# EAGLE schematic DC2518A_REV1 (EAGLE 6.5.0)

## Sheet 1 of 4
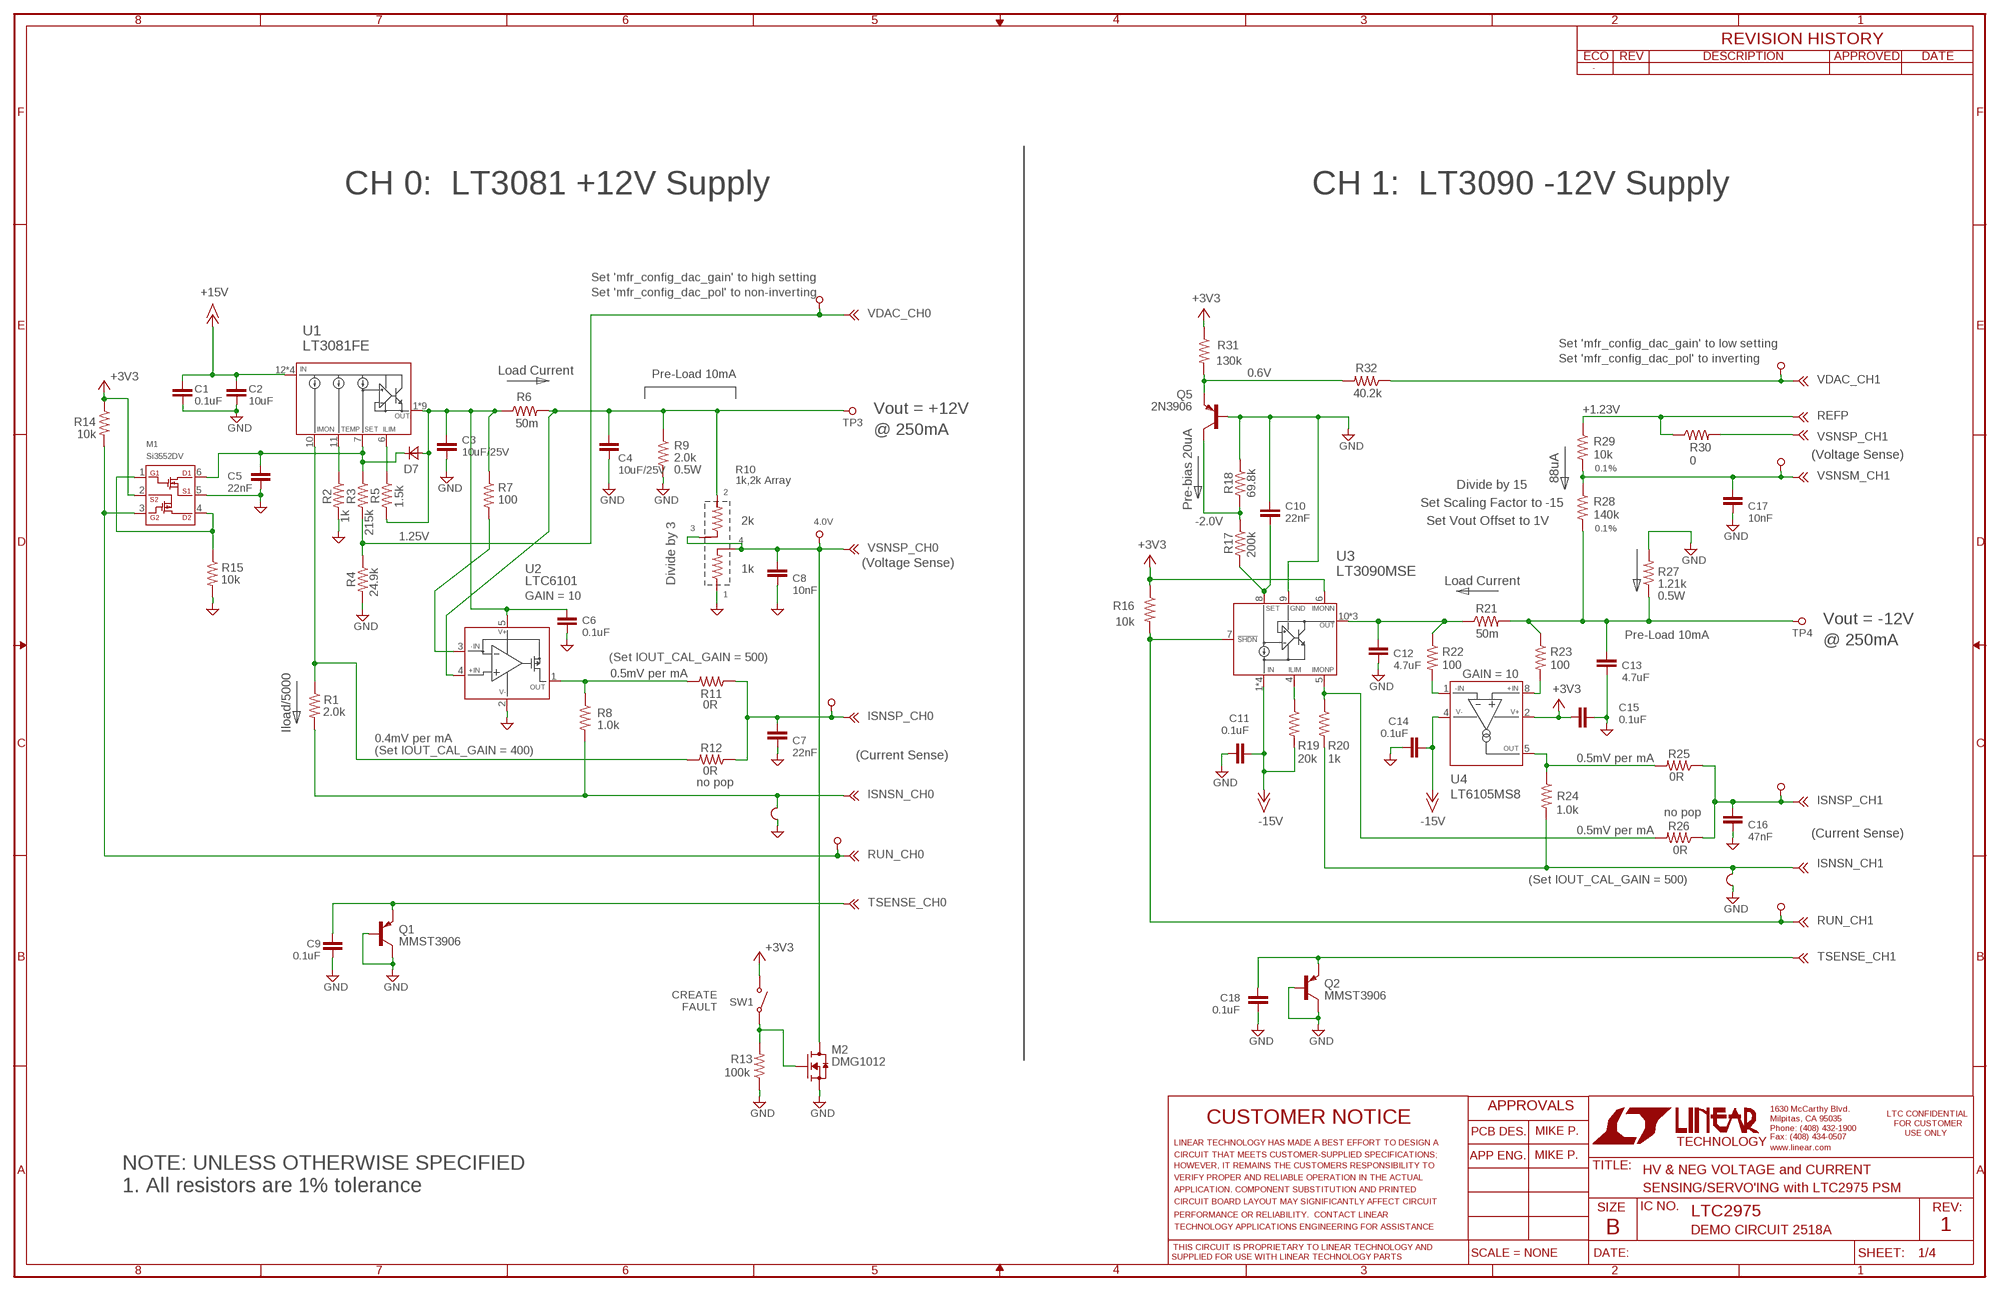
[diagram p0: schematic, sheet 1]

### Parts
C1  0.1uF  CC0603_BOX  [C0603_BOX]
C2  10uF  CC1206_BOX  [C1206_BOX]
C3  10uF/25V  CC1206_BOX  [C1206_BOX]
C4  10uF/25V  CC1206_BOX  [C1206_BOX]
C5  22nF  CC0603_BOX  [C0603_BOX]
C6  0.1uF  CC0603_BOX  [C0603_BOX]
C7  22nF  CC0603_BOX  [C0603_BOX]
C8  10nF  CC0603_BOX  [C0603_BOX]
C9  0.1uF  CC0603_BOX  [C0603_BOX]
C10  22nF  CC0603_BOX  [C0603_BOX]
C11  0.1uF  CC0603_BOX  [C0603_BOX]
C12  4.7uF  CC1206_BOX  [C1206_BOX]
C13  4.7uF  CC1206_BOX  [C1206_BOX]
C14  0.1uF  CC0603_BOX  [C0603_BOX]
C15  0.1uF  CC0603_BOX  [C0603_BOX]
C16  47nF  CC0603_BOX  [C0603_BOX]
C17  10nF  CC0603_BOX  [C0603_BOX]
C18  0.1uF  CC0603_BOX  [C0603_BOX]
D7  DIODE-SOD123  [SOD123]
M1  Si3552DV  NCH-PCH_TS  [TSOP-6]
M2  DMG1012  NCH_SOT323  [SOT323]
Q1  MMST3906  PNPSC  [SC70]
Q2  MMST3906  PNPSC  [SC70]
Q5  2N3906  PNPSOT  [SOT23]
R1  2.0k  RR0603_BOX  [R0603_BOX]
R2  1k  RR0603_BOX  [R0603_BOX]
R3  215k  RR0603_BOX  [R0603_BOX]
R4  24.9k  RR0603_BOX  [R0603_BOX]
R5  1.5k  RR0603_BOX  [R0603_BOX]
R6  50m  RR1210_BOX  [R1210_BOX]
R7  100  RR0603_BOX  [R0603_BOX]
R8  1.0k  RR0603_BOX  [R0603_BOX]
R9  2.0k  RR1210_BOX  [R1210_BOX]
R10  1k,2k Array  R_ARRAY_2X_DIVIDER  [R_ARRAY_2X_ACAS]
R11  0R  RR0603_BOX  [R0603_BOX]
R12  0R  RR0603_BOX  [R0603_BOX]
R13  100k  RR0603_BOX  [R0603_BOX]
R14  10k  RR0603_BOX  [R0603_BOX]
R15  10k  RR0603_BOX  [R0603_BOX]
R16  10k  RR0603_BOX  [R0603_BOX]
R17  200k  RR0603_BOX  [R0603_BOX]
R18  69.8k  RR0603_BOX  [R0603_BOX]
R19  20k  RR0603_BOX  [R0603_BOX]
R20  1k  RR0603_BOX  [R0603_BOX]
R21  50m  RR1210_BOX  [R1210_BOX]
R22  100  RR0603_BOX  [R0603_BOX]
R23  100  RR0603_BOX  [R0603_BOX]
R24  1.0k  RR0603_BOX  [R0603_BOX]
R25  0R  RR0603_BOX  [R0603_BOX]
R26  0R  RR0603_BOX  [R0603_BOX]
R27  1.21k  RR1210_BOX  [R1210_BOX]
R28  140k  RR0603_BOX  [R0603_BOX]
R29  10k  RR0603_BOX  [R0603_BOX]
R30  0  RR0603_BOX  [R0603_BOX]
R31  130k  RR0603_BOX  [R0603_BOX]
R32  40.2k  RR0603_BOX  [R0603_BOX]
SW1  PTS635SL25SMTR LFS  SWITCH_PTS635  [SWITCH_PTS635]
TP3  2501-2-00-80-00-00-07-0  TURRET_LARGE_2501  [TURRET_LARGE_2501]
TP4  2501-2-00-80-00-00-07-0  TURRET_LARGE_2501  [TURRET_LARGE_2501]
TP15  TESTPOINT  [VIA]
TP16  TESTPOINT  [VIA]
TP17  TESTPOINT  [VIA]
TP18  TESTPOINT  [VIA]
TP19  TESTPOINT  [VIA]
TP20  TESTPOINT  [VIA]
TP27  TESTPOINT  [VIA]
TP28  TESTPOINT  [VIA]
U1  LT3081FE  [TSSOP16EXP]
U2  LTC6101  [TSOT23-5]
U3  LT3090MSE  [MSOP12_EXP]
U4  LT6105MS8  [MSOP8]
U$39  KELVIN-CONNECT  [KELVIN]
U$40  KELVIN-CONNECT  [KELVIN]

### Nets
+3V3: C15.1 M1.2(S2) R14.1 R16.1 R31.1 SW1.SW1 U3.6(IMONN) U4.2(V+) ; also sheet 2,3,4
+15V: C1.1 C2.1 U1.12(IN) U1.13(IN) U1.14(IN) U1.15(IN) ; also sheet 4
-15V: C11.1 C14.1 R19.2 U3.1(IN) U3.2(IN) U3.3(IN) U3.PAD(IN) U4.4(V-) ; also sheet 4
GND: C1.2 C2.2 C3.2 C4.2 C5.2 C6.2 C7.2 C8.2 C9.2 C10.1 C11.2 C12.2 C13.2 C14.2 C15.2 C16.2 C17.2 C18.2 M1.5(S1) M2.2(S) Q1.1(B) Q1.3(C) Q2.1(B) Q2.3(C) Q5.1(B) R2.2 R4.2 R9.2 R10.P$1 R13.1 R15.2 R18.1 R27.2 U2.2(V-) U3.9(GND) U$39.P$1 U$40.P$1 ; also sheet 2,3,4
ISNSN_CH0 [GNDsns]: R1.2 R8.2 U$40.P$2 ; also sheet 3
ISNSN_CH1: R20.2 R24.2 U$39.P$2 ; also sheet 3
ISNSP_CH0: C7.1 R11.1 R12.1 TP27.1 ; also sheet 3
ISNSP_CH1: C16.1 R25.1 R26.1 TP28.1 ; also sheet 3
N$3: C3.1 C6.1 D7.A R5.2 R6.1 R7.1 U1.1(OUT) U1.2(OUT) U1.3(OUT) U1.4(OUT) U1.5(OUT) U1.8(OUT) U1.9(OUT) U1.16(OUT) U1.EXP(OUT) U2.5(V+)
N$5: R5.1 U1.6(ILIM)
N$6: R2.1 U1.11(TEMP)
N$7: R1.1 R12.2 U1.10(IMON)
N$8: C4.1 R6.2 R9.1 R10.P$2 TP3.TP U2.4(+IN)
N$10: R8.1 R11.2 U2.1(OUT)
N$11: C10.2 R17.2 U3.8(SET)
N$12: Q5.3(C) R17.1 R18.2
N$13: C12.1 R21.1 R22.1 U3.10(OUT) U3.11(OUT) U3.12(OUT)
N$14: C13.1 R21.2 R23.1 R27.1 R28.2 TP4.TP
N$15: R22.2 U4.1(-IN)
N$17: R20.1 R26.2 U3.5(IMONP)
N$18: R23.2 U4.8(+IN)
N$19: R24.1 R25.2 U4.5(OUT)
N$21: Q5.2(E) R31.2 R32.2
N$27: R19.1 U3.4(ILIM)
N$30: M2.1(G) R13.2 SW1.SW2
N$63: C5.1 D7.C M1.6(D1) R3.1 U1.7(SET)
N$70: R7.2 U2.3(-IN)
N$71: M1.1(G1) M1.4(D2) R15.1
REFP: R29.1 R30.1 ; also sheet 2,3
RUN_CH0: M1.3(G2) R14.2 TP15.1 ; also sheet 3
RUN_CH1: R16.2 TP20.1 U3.7(SHDN) ; also sheet 3
TSENSE_CH0: C9.1 Q1.2(E) ; also sheet 3
TSENSE_CH1: C18.1 Q2.2(E) ; also sheet 3
VDAC_CH0: R3.2 R4.1 TP16.1 ; also sheet 3
VDAC_CH1: R32.1 TP18.1 ; also sheet 3
VSNSM_CH1: C17.1 R28.1 R29.2 TP19.1 ; also sheet 3
VSNSP_CH0: C8.1 M2.3(D) R10.P$3 R10.P$4 TP17.1 ; also sheet 3
VSNSP_CH1: R30.2 ; also sheet 3

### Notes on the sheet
- CH 0:  LT3081 +12V Supply | CH 1:  LT3090 -12V Supply
- Set 'mfr_config_dac_gain' to high setting
- Set 'mfr_config_dac_pol' to non-inverting
- Set 'mfr_config_dac_gain' to low setting
- Set 'mfr_config_dac_pol' to inverting
- Load Current | 0.6V
- Pre-Load 10mA
- Vout = +12V | +1.23V
- @ 250mA
- (Voltage Sense)
- 0.5W | 0.1%
- 88uA
- Divide by 15
- Pre-bias 20uA | Set Scaling Factor to -15
- 2k | 4.0V | -2.0V | Set Vout Offset to 1V
- 0.1%
- 1.25V
- (Voltage Sense)
- 1k
- Divide by 3 | Load Current
- GAIN = 10 | 0.5W
- Vout = -12V
- Pre-Load 10mA
- @ 250mA
- (Set IOUT_CAL_GAIN = 500)
- 0.5mV per mA | GAIN = 10
- Iload/5000
- 0.4mV per mA
- (Set IOUT_CAL_GAIN = 400)
- (Current Sense) | 0.5mV per mA
- no pop
- no pop
- 0.5mV per mA | (Current Sense)
- (Set IOUT_CAL_GAIN = 500)
- CREATE
   FAULT
- MIKE P.
- MIKE P.
- HV & NEG VOLTAGE and CURRENT
- NOTE: UNLESS OTHERWISE SPECIFIED
  1. All resistors are 1% tolerance
- SENSING/SERVO'ING with LTC2975 PSM
- LTC2975
- DEMO CIRCUIT 2518A | 1

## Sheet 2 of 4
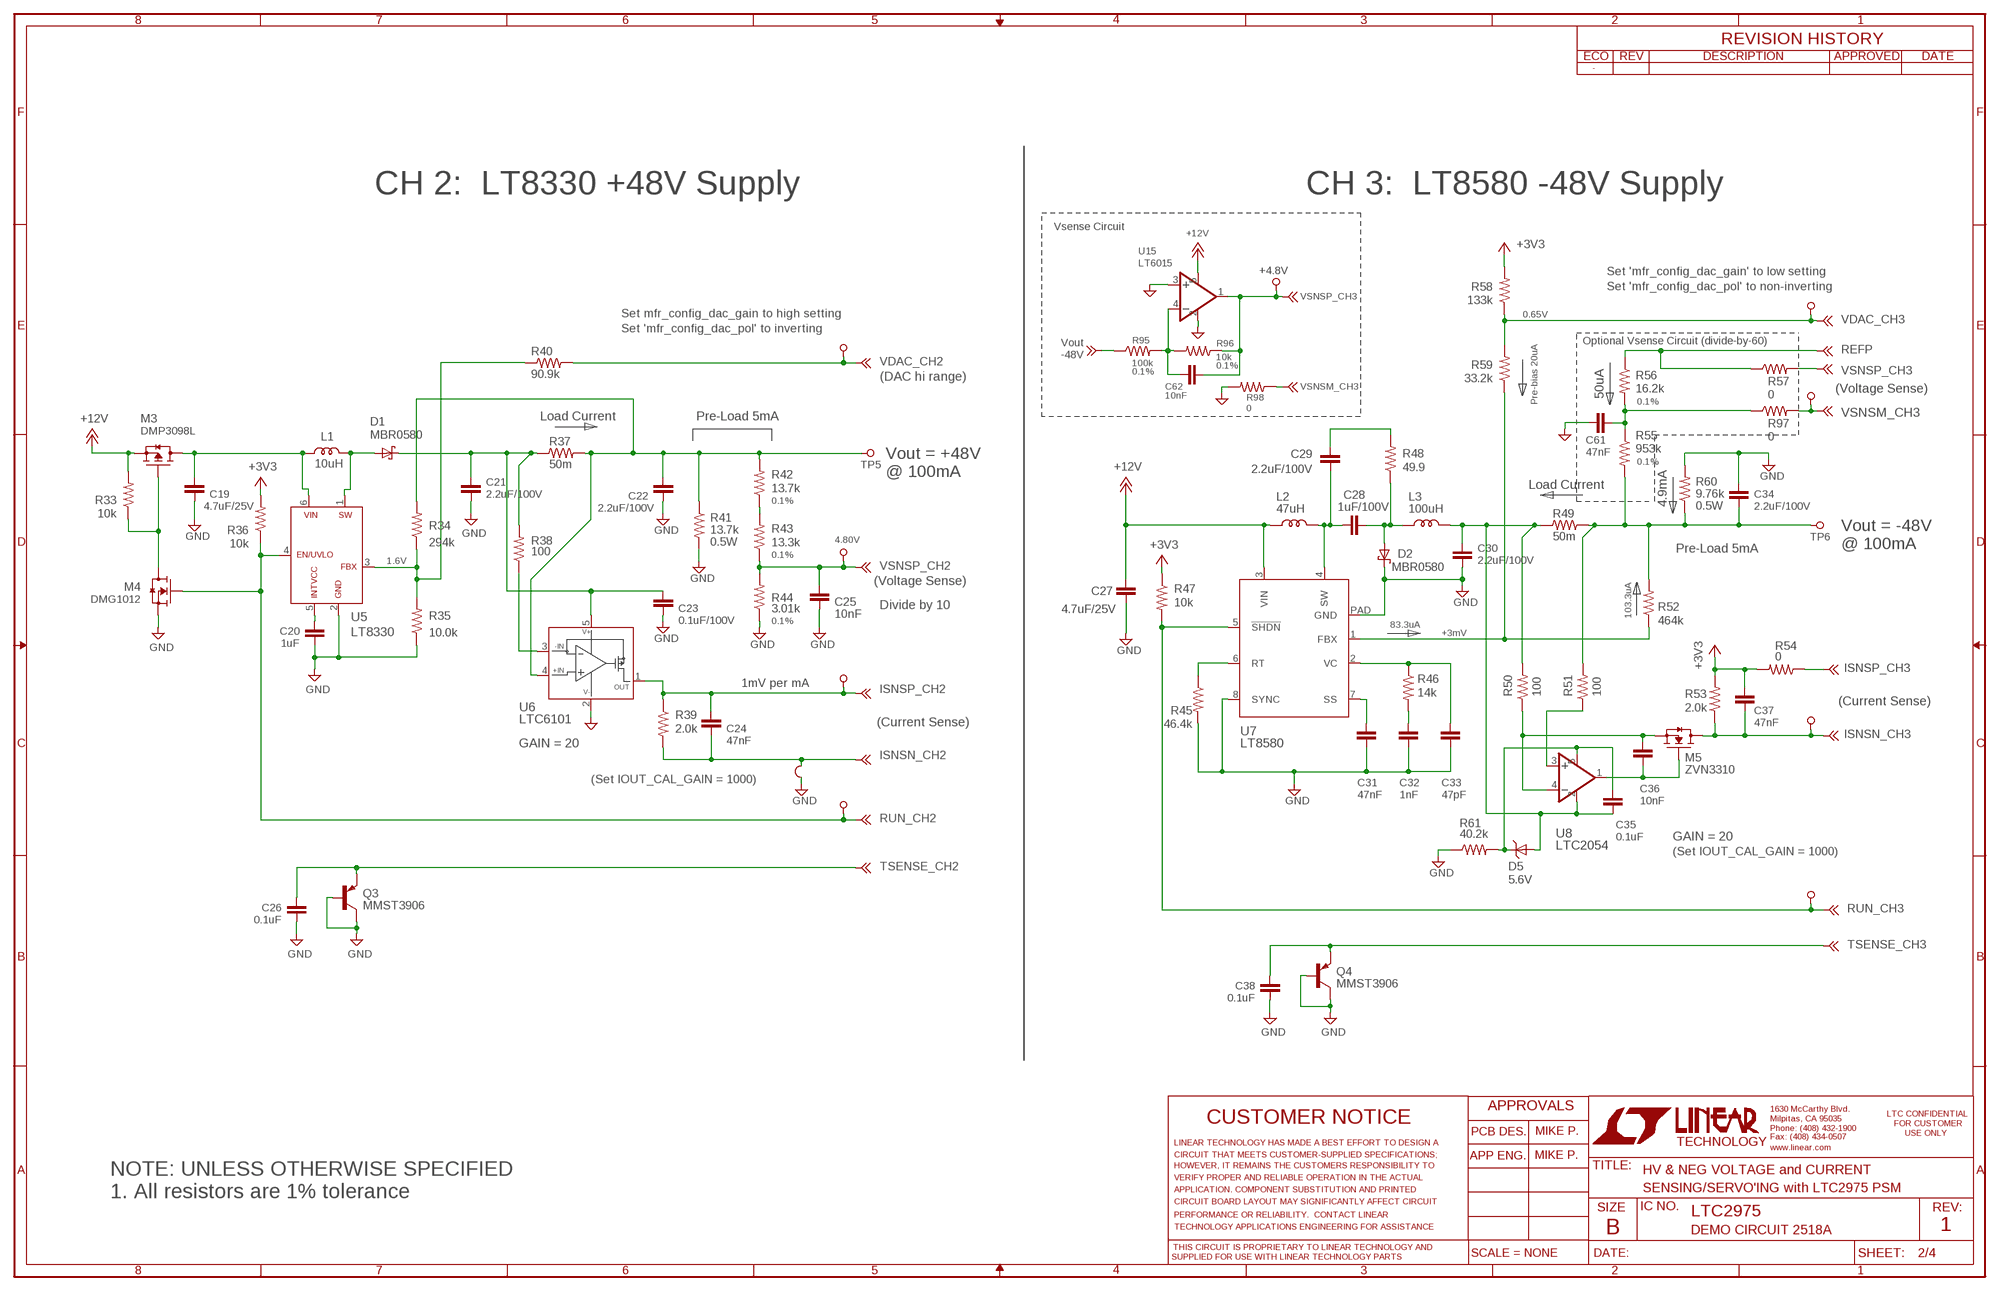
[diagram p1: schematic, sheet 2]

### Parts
C19  4.7uF/25V  CC0805_BOX  [C0805_BOX]
C20  1uF  CC0603_BOX  [C0603_BOX]
C21  2.2uF/100V  CC1210_BOX  [C1210_BOX]
C22  2.2uF/100V  CC1210_BOX  [C1210_BOX]
C23  0.1uF/100V  CC0603_BOX  [C0603_BOX]
C24  47nF  CC0603_BOX  [C0603_BOX]
C25  10nF  CC0603_BOX  [C0603_BOX]
C26  0.1uF  CC0603_BOX  [C0603_BOX]
C27  4.7uF/25V  CC1206_BOX  [C1206_BOX]
C28  1uF/100V  CC0805_BOX  [C0805_BOX]
C29  2.2uF/100V  CC1206_BOX  [C1206_BOX]
C30  2.2uF/100V  CC1210_BOX  [C1210_BOX]
C31  47nF  CC0603_BOX  [C0603_BOX]
C32  1nF  CC0603_BOX  [C0603_BOX]
C33  47pF  CC0603_BOX  [C0603_BOX]
C34  2.2uF/100V  CC1210_BOX  [C1210_BOX]
C35  0.1uF  CC0603_BOX  [C0603_BOX]
C36  10nF  CC0603_BOX  [C0603_BOX]
C37  47nF  CC0603_BOX  [C0603_BOX]
C38  0.1uF  CC0603_BOX  [C0603_BOX]
C61  47nF  CC0402  [C0402_BOX]
C62  10nF  CC0402  [C0402_BOX]
D1  MBR0580  SCHOTTKY-DIODESOD123FL  [SOD123FL]
D2  MBR0580  SCHOTTKY-DIODESOD123FL  [SOD123FL]
D5  5.6V  ZENER-DIODESOD123  [SOD123]
L1  10uH  WE-MAPI-3015  [WE-MAPI-3015]
L2  47uH  WE-LQS-4018  [WE-LQS-4018]
L3  100uH  WE-LQS-4018  [WE-LQS-4018]
M3  DMP3098L  PCH_SOT23  [SOT23]
M4  DMG1012  NCH_SOT323  [SOT323]
M5  ZVN3310  NCH_SOT23  [SOT23]
Q3  MMST3906  PNPSC  [SC70]
Q4  MMST3906  PNPSC  [SC70]
R33  10k  RR0603_BOX  [R0603_BOX]
R34  294k  RR0603_BOX  [R0603_BOX]
R35  10.0k  RR0603_BOX  [R0603_BOX]
R36  10k  RR0603_BOX  [R0603_BOX]
R37  50m  RR1210_BOX  [R1210_BOX]
R38  100  RR0603_BOX  [R0603_BOX]
R39  2.0k  RR0603_BOX  [R0603_BOX]
R40  90.9k  RR0603_BOX  [R0603_BOX]
R41  13.7k  RR1210_BOX  [R1210_BOX]
R42  13.7k  RR0603_BOX  [R0603_BOX]
R43  13.3k  RR0603_BOX  [R0603_BOX]
R44  3.01k  RR0603_BOX  [R0603_BOX]
R45  46.4k  RR0402_BOX  [R0402_BOX]
R46  14k  RR0603_BOX  [R0603_BOX]
R47  10k  RR0603_BOX  [R0603_BOX]
R48  49.9  RR0603_BOX  [R0603_BOX]
R49  50m  RR1210_BOX  [R1210_BOX]
R50  100  RR0603_BOX  [R0603_BOX]
R51  100  RR0603_BOX  [R0603_BOX]
R52  464k  RR0603_BOX  [R0603_BOX]
R53  2.0k  RR0603_BOX  [R0603_BOX]
R54  0  RR0402_BOX  [R0402_BOX]
R55  953k  RR0402_BOX  [R0402_BOX]
R56  16.2k  RR0402_BOX  [R0402_BOX]
R57  0  RR0402_BOX  [R0402_BOX]
R58  133k  RR0402_BOX  [R0402_BOX]
R59  33.2k  RR0402_BOX  [R0402_BOX]
R60  9.76k  RR1210_BOX  [R1210_BOX]
R61  40.2k  RR0603_BOX  [R0603_BOX]
R95  100k  RR0402_BOX  [R0402_BOX]
R96  10k  RR0402_BOX  [R0402_BOX]
R97  0  RR0402_BOX  [R0402_BOX]
R98  0  RR0402_BOX  [R0402_BOX]
TP5  2501-2-00-80-00-00-07-0  TURRET_LARGE_2501  [TURRET_LARGE_2501]
TP6  2501-2-00-80-00-00-07-0  TURRET_LARGE_2501  [TURRET_LARGE_2501]
TP21  TESTPOINT  [VIA]
TP22  TESTPOINT  [VIA]
TP23  TESTPOINT  [VIA]
TP24  TESTPOINT  [VIA]
TP25  TESTPOINT  [VIA]
TP26  TESTPOINT  [VIA]
TP29  TESTPOINT  [VIA]
TP30  TESTPOINT  [VIA]
TP31  TESTPOINT  [VIA]
U5  LT8330  [TSOT23-6]
U6  LTC6101  [TSOT23-5]
U7  LT8580  [MSOP8_EXP]
U8  LTC2054  [TSOT23-5]
U15  LT6015  [TSOT23-5]
U$41  KELVIN-CONNECT  [KELVIN]

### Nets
+3V3: C37.1 R36.2 R47.1 R53.2 R54.2 R58.2 ; also sheet 1,3,4
+12V: C27.1 L2.1 M3.2(S) R33.2 U7.3(VIN) U15.5(V+) ; also sheet 4
GND: C19.2 C20.2 C21.2 C22.2 C23.2 C25.2 C26.2 C27.2 C30.2 C31.2 C32.2 C33.2 C34.1 C38.2 C61.2 D2.C M4.2(S) Q3.1(B) Q3.3(C) Q4.1(B) Q4.3(C) R35.1 R41.2 R44.1 R45.2 R60.2 R61.1 R98.2 U5.2(GND) U6.2(V-) U7.8(SYNC) U7.PAD(GND) U15.2(V-) U15.3(+IN) U$41.P$1 ; also sheet 1,3,4
ISNSN_CH2: C24.2 R39.2 U$41.P$2 ; also sheet 3
ISNSN_CH3: C37.2 M5.3(D) R53.1 TP30.1 ; also sheet 3
ISNSP_CH2: C24.1 R39.1 TP29.1 U6.1(OUT) ; also sheet 3
ISNSP_CH3: R54.1 ; also sheet 3
N$2: R42.1 R43.2
N$9 [HV]: R38.1 U6.3(-IN)
N$20: R34.1 R35.2 R40.1 U5.3(FBX)
N$22: C20.1 U5.5(INTVCC)
N$23 [HV]: C21.1 C23.1 D1.C R37.1 R38.2 U6.5(V+)
N$24 [HV]: C30.1 C35.2 D5.A L3.2 R49.1 R50.2 U8.2(V-)
N$26 [HV]: D1.A L1.2 U5.1(SW)
N$28 [HV]: C34.2 R49.2 R51.2 R52.2 R55.2 R60.1 R95.1 TP6.TP
N$29 [HV]: C22.1 R34.2 R37.2 R41.1 R42.2 TP5.TP U6.4(+IN)
N$31: R45.1 U7.6(RT)
N$32: C19.1 L1.1 M3.3(D) U5.6(VIN)
N$33: C31.1 U7.7(SS)
N$34: C32.1 R46.2
N$35: C33.1 R46.1 U7.2(VC)
N$36: R52.1 R59.1 U7.1(FBX)
N$37 [HV]: C28.1 C29.2 L2.2 U7.4(SW)
N$39 [HV]: C28.2 D2.A L3.1 R48.1
N$56 [HV]: C29.1 R48.2
N$57 [HV]: R51.1 U8.3(+IN)
N$60 [HV]: C35.1 D5.C R61.2 U8.5(V+)
N$61 [HV]: C36.1 M5.2(S) R50.1 U8.4(-IN)
N$62 [HV]: C36.2 M5.1(G) U8.1(OUT)
N$72: M3.1(G) M4.3(D) R33.1
N$75: C62.2 R95.2 R96.2 U15.4(-IN)
N$77: C61.1 R55.1 R56.2 R97.1
REFP: R56.1 R57.1 ; also sheet 1,3
RUN_CH2: M4.1(G) R36.1 TP23.1 U5.4(EN/UVLO) ; also sheet 3
RUN_CH3: R47.2 TP26.1 U7.5(!SHDN) ; also sheet 3
TSENSE_CH2: C26.1 Q3.2(E) ; also sheet 3
TSENSE_CH3: C38.1 Q4.2(E) ; also sheet 3
VDAC_CH2: R40.2 TP21.1 ; also sheet 3
VDAC_CH3: R58.1 R59.2 TP24.1 ; also sheet 3
VSNSM_CH3: R97.2 R98.1 TP25.1 ; also sheet 3
VSNSP_CH2: C25.1 R43.1 R44.2 TP22.1 ; also sheet 3
VSNSP_CH3: C62.1 R57.2 R96.1 TP31.1 U15.1(OUT) ; also sheet 3

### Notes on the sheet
- CH 2:  LT8330 +48V Supply | CH 3:  LT8580 -48V Supply
- Vsense Circuit
- +4.8V
- Set 'mfr_config_dac_gain' to low setting
- Set 'mfr_config_dac_pol' to non-inverting
- Set mfr_config_dac_gain to high setting | 0.65V
- Set 'mfr_config_dac_pol' to inverting
- Vout
  -48V
- Optional Vsense Circuit (divide-by-60)
- 0.1%
- 0.1%
- (DAC hi range)
- (Voltage Sense)
- 50uA
- Pre-bias 20uA | 0.1%
- Load Current | Pre-Load 5mA
- Vout = +48V
- 0.1%
- @ 100mA
- Load Current
- 0.1%
- 4.9mA | 0.5W
- Vout = -48V
- 4.80V
- 0.5W | @ 100mA
- Pre-Load 5mA
- 0.1%
- 1.6V
- 103.3uA
- (Voltage Sense)
- Divide by 10
- 83.3uA
- 0.1%
- +3mV
- 1mV per mA
- (Current Sense)
- (Current Sense)
- GAIN = 20
- (Set IOUT_CAL_GAIN = 1000)
- GAIN = 20
- (Set IOUT_CAL_GAIN = 1000)
- MIKE P.
- MIKE P.
- HV & NEG VOLTAGE and CURRENT
- SENSING/SERVO'ING with LTC2975 PSM
- NOTE: UNLESS OTHERWISE SPECIFIED
  1. All resistors are 1% tolerance
- LTC2975
- DEMO CIRCUIT 2518A | 1

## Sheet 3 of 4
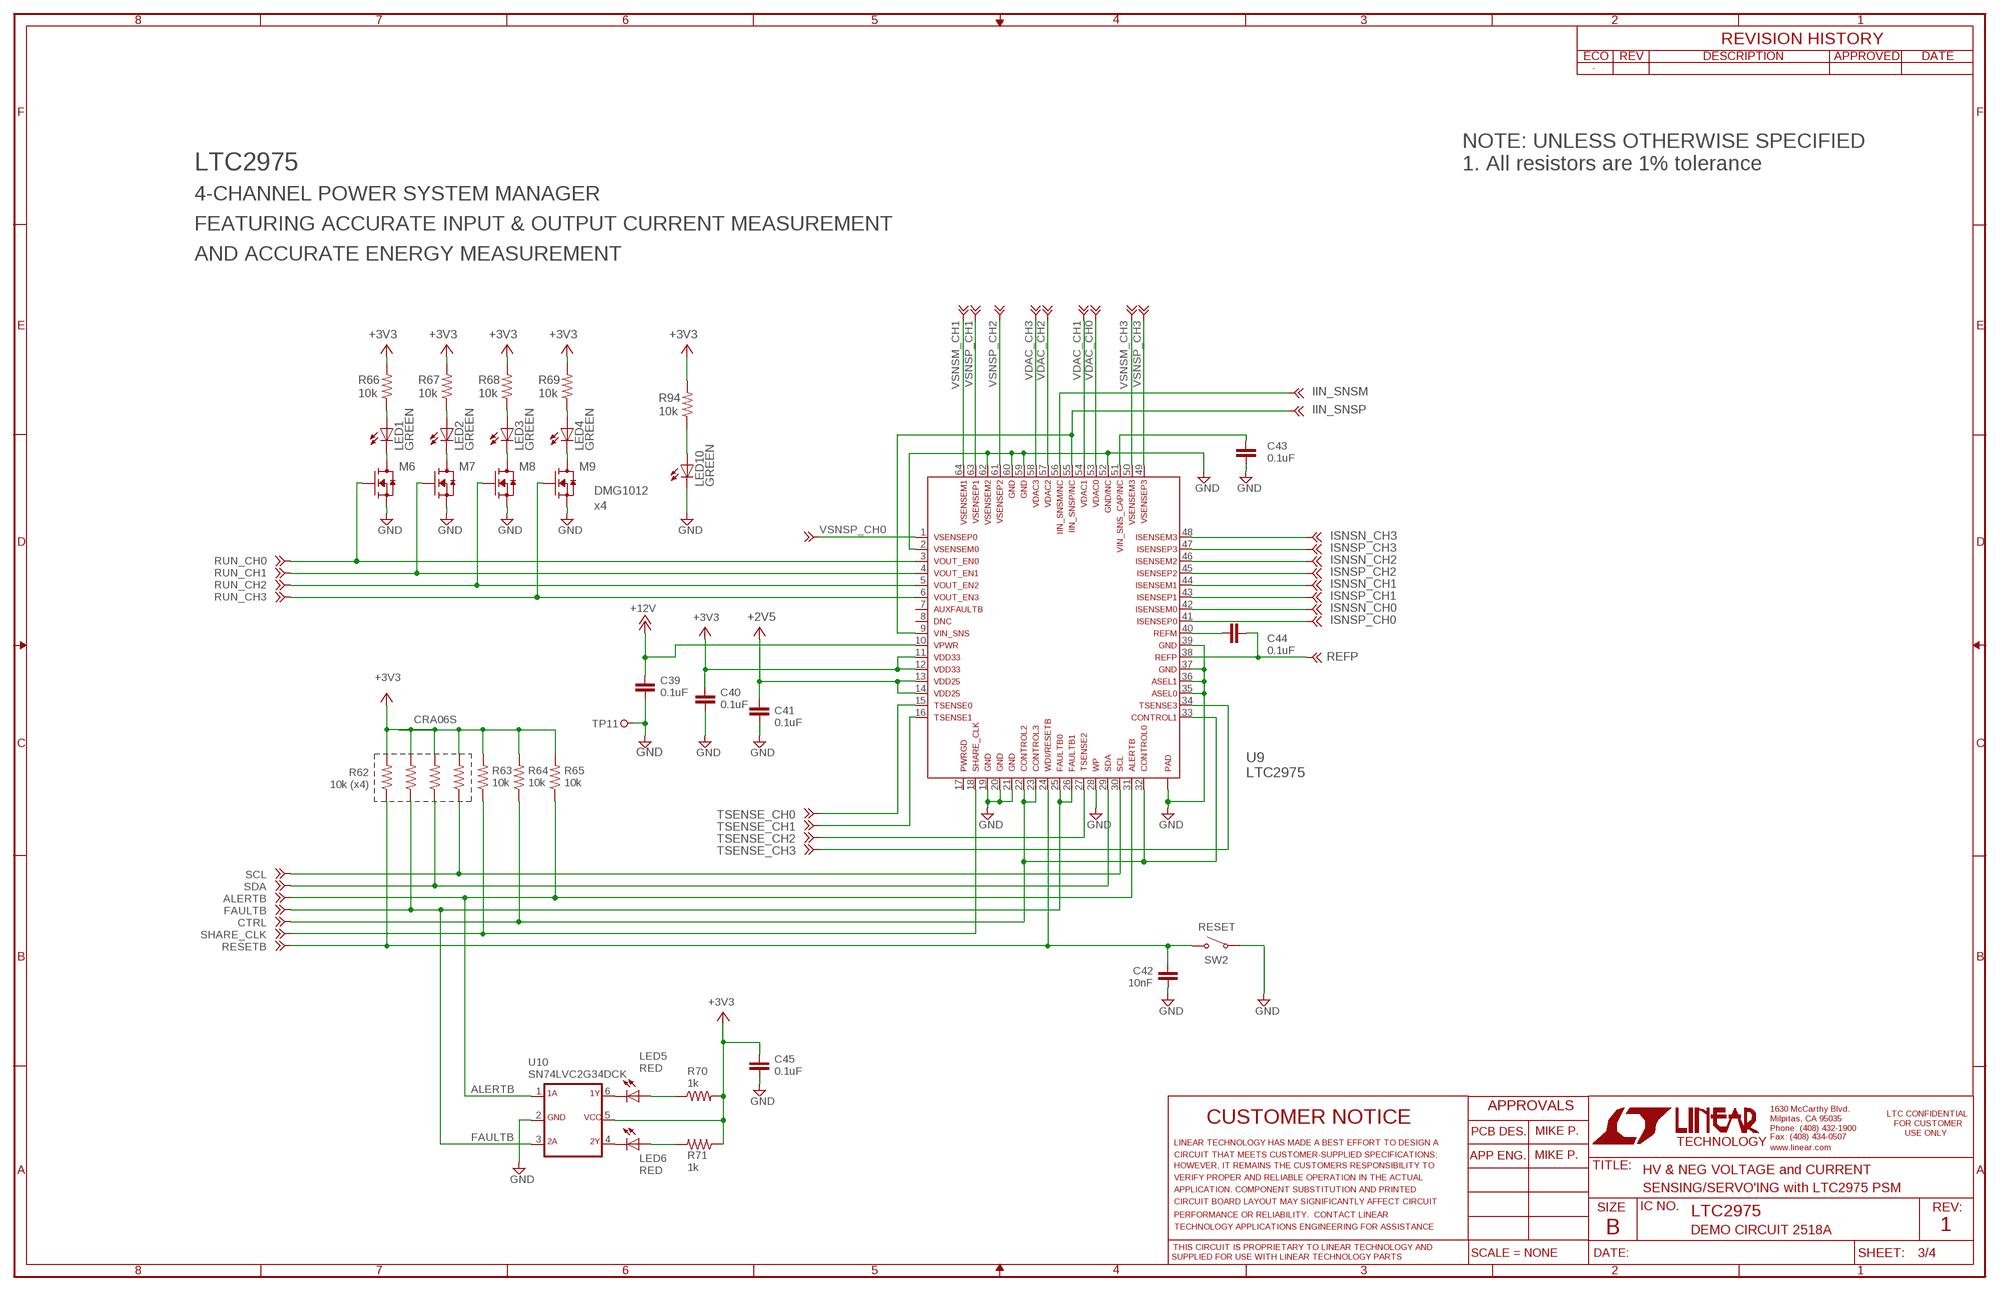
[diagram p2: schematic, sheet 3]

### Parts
C39  0.1uF  CC0603_BOX  [C0603_BOX]
C40  0.1uF  CC0603_BOX  [C0603_BOX]
C41  0.1uF  CC0603_BOX  [C0603_BOX]
C42  10nF  CC0603_BOX  [C0603_BOX]
C43  0.1uF  CC0603_BOX  [C0603_BOX]
C44  0.1uF  CC0603_BOX  [C0603_BOX]
C45  0.1uF  CC0603_BOX  [C0603_BOX]
LED1  GREEN  LED0603  [0603]
LED2  GREEN  LED0603  [0603]
LED3  GREEN  LED0603  [0603]
LED4  GREEN  LED0603  [0603]
LED5  RED  LED0603  [0603]
LED6  RED  LED0603  [0603]
LED10  GREEN  LED0603  [0603]
M6  DMG1012  NCH_SOT323  [SOT323]
M7  DMG1012  NCH_SOT323  [SOT323]
M8  DMG1012  NCH_SOT323  [SOT323]
M9  DMG1012  NCH_SOT323  [SOT323]
R62  10k (x4)  R_ARRAY_4X_CRA06S  [R_VISHAY_CRA06S]
R63  10k  RR0603_BOX  [R0603_BOX]
R64  10k  RR0603_BOX  [R0603_BOX]
R65  10k  RR0603_BOX  [R0603_BOX]
R66  10k  RR0603_BOX  [R0603_BOX]
R67  10k  RR0603_BOX  [R0603_BOX]
R68  10k  RR0603_BOX  [R0603_BOX]
R69  10k  RR0603_BOX  [R0603_BOX]
R70  1k  RR0603_BOX  [R0603_BOX]
R71  1k  RR0603_BOX  [R0603_BOX]
R94  10k  RR0603_BOX  [R0603_BOX]
SW2  PTS635SL25SMTR LFS  SWITCH_PTS635  [SWITCH_PTS635]
TP11  2501-2-00-80-00-00-07-0  TURRET_LARGE_2501  [TURRET_LARGE_2501]
U9  LTC2975  [QFN64_9X9]
U10  SN74LVC2G34DCK  [SC70-6]

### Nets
+2V5: C41.1 U9.13 U9.14
+3V3: C40.1 C45.1 R62.R1_2 R62.R2_2 R62.R3_2 R62.R4_2 R63.2 R64.2 R65.2 R66.2 R67.2 R68.2 R69.2 R70.2 R71.1 R94.2 U9.11 U9.12 U10.5 ; also sheet 1,2,4
+12V_IN: C39.1 U9.10 ; supply symbol labelled +12V ; also sheet 4
ALERTB: R65.1 U9.31 U10.1 ; also sheet 4
CTRL: R64.1 U9.22 U9.23 U9.32 U9.33 ; also sheet 4
FAULTB: R62.R2_1 U9.25 U9.26 U10.3 ; also sheet 4
GND: C39.2 C40.2 C41.2 C42.2 C43.2 C45.2 LED10.C M6.2(S) M7.2(S) M8.2(S) M9.2(S) SW2.SW2 TP11.TP U9.2 U9.19 U9.20 U9.21 U9.28 U9.35 U9.36 U9.37 U9.39 U9.52 U9.59 U9.60 U9.62 U9.PAD U10.2 ; also sheet 1,2,4
IIN_SNSM: U9.56 ; also sheet 4
IIN_SNSP: U9.9 U9.55 ; also sheet 4
ISNSN_CH0 [GNDsns]: U9.42 ; also sheet 1
ISNSN_CH1: U9.44 ; also sheet 1
ISNSN_CH2: U9.46 ; also sheet 2
ISNSN_CH3: U9.48 ; also sheet 2
ISNSP_CH0: U9.41 ; also sheet 1
ISNSP_CH1: U9.43 ; also sheet 1
ISNSP_CH2: U9.45 ; also sheet 2
ISNSP_CH3: U9.47 ; also sheet 2
N$1: C43.1 U9.51
N$25: LED1.A R66.1
N$38: LED1.C M6.3(D)
N$40: LED2.A R67.1
N$41: LED2.C M7.3(D)
N$43: LED3.A R68.1
N$45: LED3.C M8.3(D)
N$49: LED4.A R69.1
N$53: C44.1 U9.40
N$58: LED4.C M9.3(D)
N$64: LED5.A R70.1
N$65: LED6.A R71.2
N$67: LED6.C U10.4
N$68: LED5.C U10.6
N$73: LED10.A R94.1
REFP: C44.2 U9.38 ; also sheet 1,2
RESETB: C42.1 R62.R1_1 SW2.SW1 U9.24 ; also sheet 4
RUN_CH0: M6.1(G) U9.3 ; also sheet 1
RUN_CH1: M7.1(G) U9.4 ; also sheet 1
RUN_CH2: M8.1(G) U9.5 ; also sheet 2
RUN_CH3: M9.1(G) U9.6 ; also sheet 2
SCL: R62.R4_1 U9.30 ; also sheet 4
SDA: R62.R3_1 U9.29 ; also sheet 4
SHARE_CLK: R63.1 U9.18 ; also sheet 4
TSENSE_CH0: U9.15 ; also sheet 1
TSENSE_CH1: U9.16 ; also sheet 1
TSENSE_CH2: U9.27 ; also sheet 2
TSENSE_CH3: U9.34 ; also sheet 2
VDAC_CH0: U9.53 ; also sheet 1
VDAC_CH1: U9.54 ; also sheet 1
VDAC_CH2: U9.57 ; also sheet 2
VDAC_CH3: U9.58 ; also sheet 2
VSNSM_CH1: U9.64 ; also sheet 1
VSNSM_CH3: U9.50 ; also sheet 2
VSNSP_CH0: U9.1 ; also sheet 1
VSNSP_CH1: U9.63 ; also sheet 1
VSNSP_CH2: U9.61 ; also sheet 2
VSNSP_CH3: U9.49 ; also sheet 2
Unconnected: U9.7 U9.8 U9.17

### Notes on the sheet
- LTC2975
- NOTE: UNLESS OTHERWISE SPECIFIED
  1. All resistors are 1% tolerance
- 4-CHANNEL POWER SYSTEM MANAGER
- FEATURING ACCURATE INPUT & OUTPUT CURRENT MEASUREMENT
- AND ACCURATE ENERGY MEASUREMENT
- x4
- CRA06S
- RESET
- MIKE P.
- MIKE P.
- HV & NEG VOLTAGE and CURRENT
- SENSING/SERVO'ING with LTC2975 PSM
- LTC2975
- DEMO CIRCUIT 2518A | 1

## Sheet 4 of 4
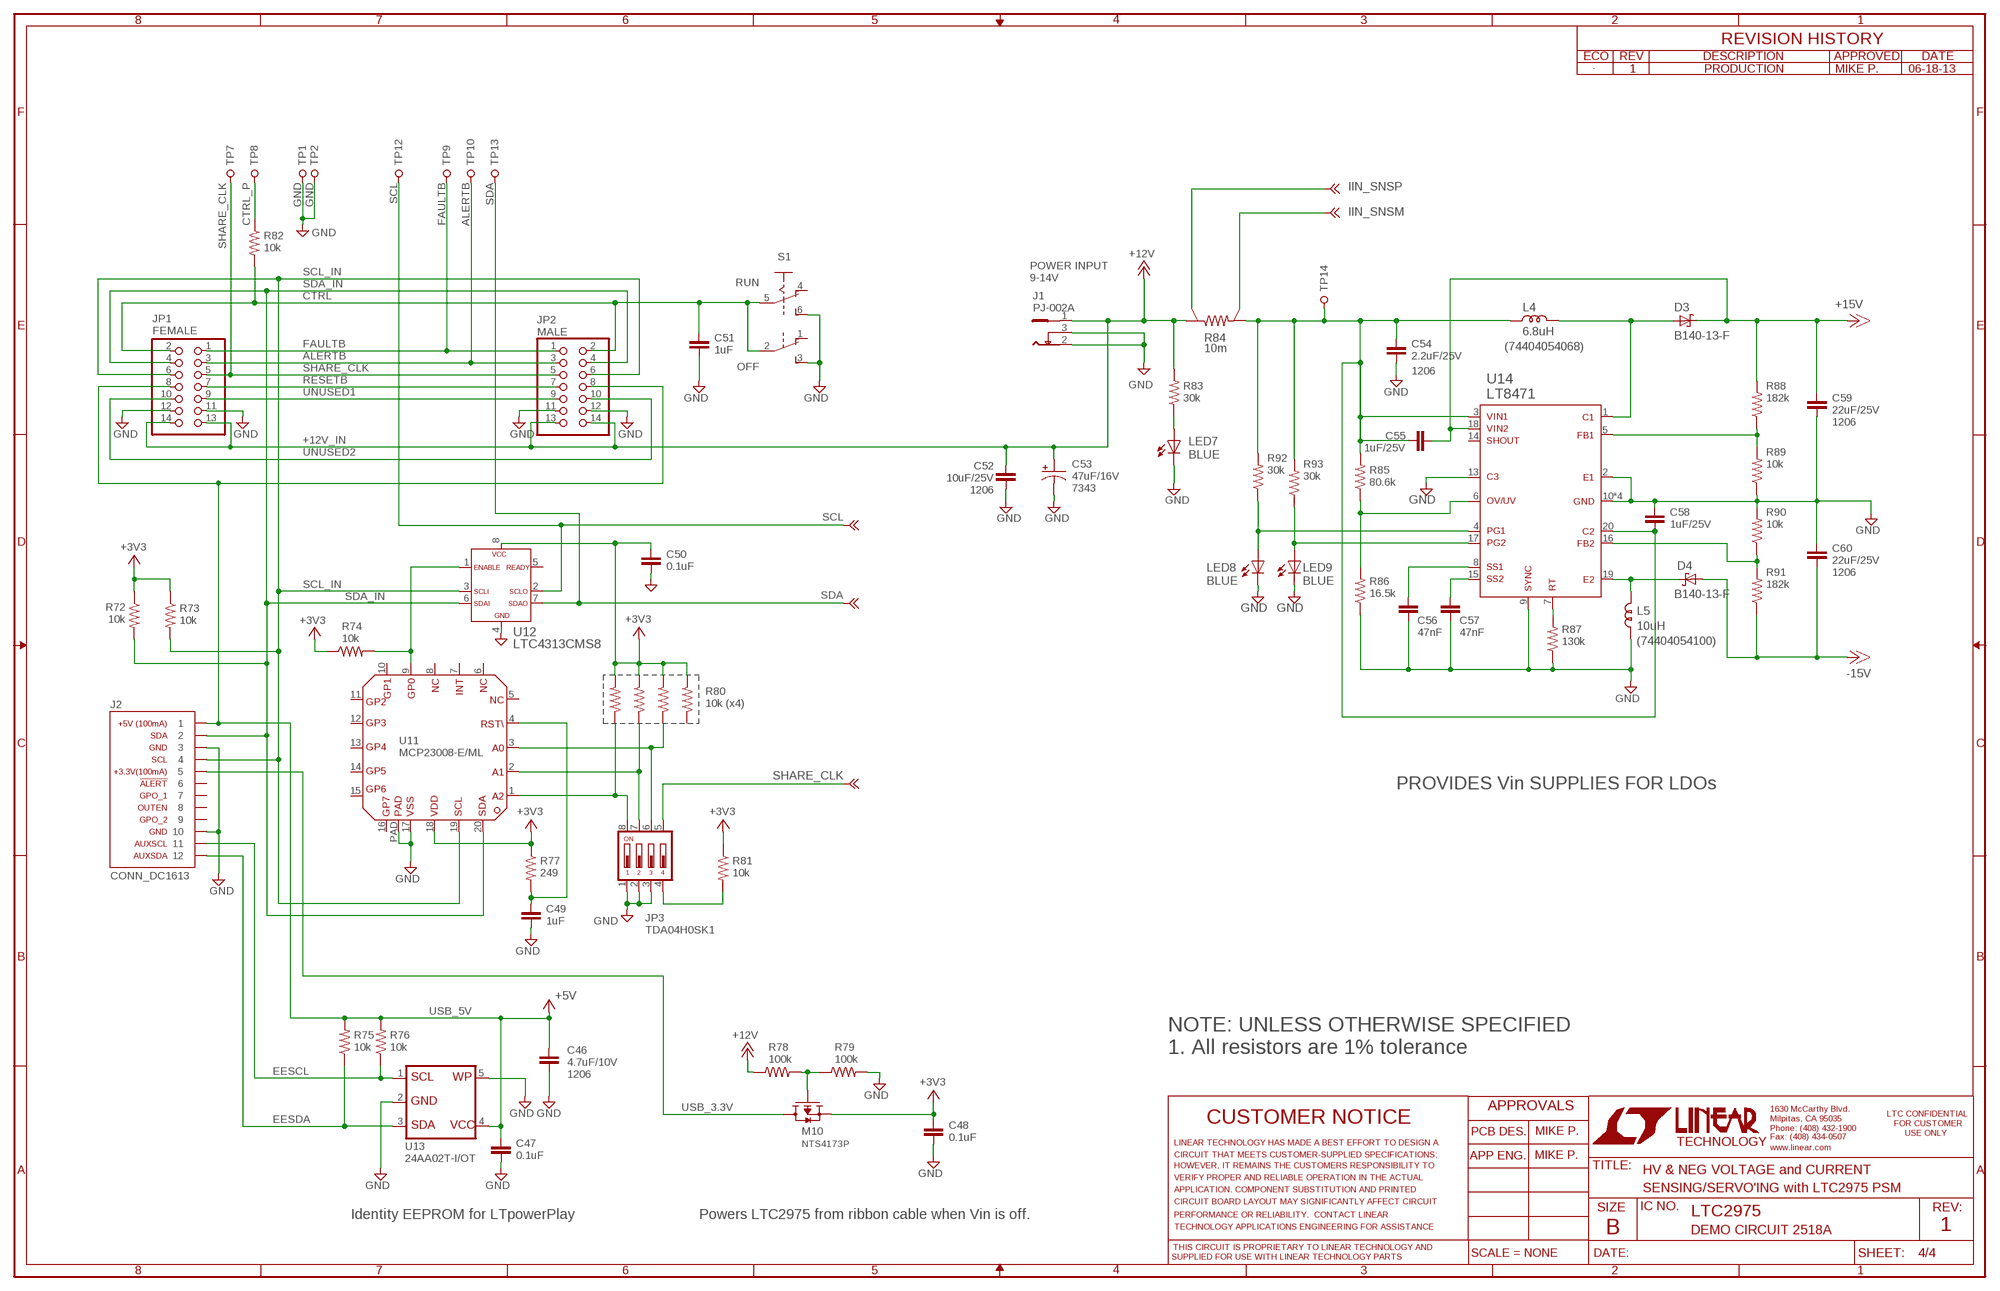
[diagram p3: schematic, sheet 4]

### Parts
C46  4.7uF/10V  CC1206_BOX  [C1206_BOX]
C47  0.1uF  CC0603_BOX  [C0603_BOX]
C48  0.1uF  CC0603_BOX  [C0603_BOX]
C49  1uF  CC0603_BOX  [C0603_BOX]
C50  0.1uF  CC0603_BOX  [C0603_BOX]
C51  1uF  CC0603_BOX  [C0603_BOX]
C52  10uF/25V  CC1206_BOX  [C1206_BOX]
C53  47uF/16V  CPOL-US7343  [C7343]
C54  2.2uF/25V  CC1206_BOX  [C1206_BOX]
C55  1uF/25V  CC1206_BOX  [C1206_BOX]
C56  47nF  CC0603_BOX  [C0603_BOX]
C57  47nF  CC0603_BOX  [C0603_BOX]
C58  1uF/25V  CC0805_BOX  [C0805_BOX]
C59  22uF/25V  CC1206_BOX  [C1206_BOX]
C60  22uF/25V  CC1206_BOX  [C1206_BOX]
D3  B140-13-F  SCHOTTKY-DIODESMA  [SMA]
D4  B140-13-F  SCHOTTKY-DIODESMA  [SMA]
J1  PJ-002A  [PJ-002A]
J2  CONN_DC1613  [CONN_DC1613]
JP1  FEMALE  PINHD-2X07_2.00  [2X07M]
JP2  MALE  PINHD-2X07_2.00  [2X07M]
JP3  TDA04H0SK1  [SMT_DIP_4]
L4  6.8uH  WE-LQS-5040  [WE-LQS-5040]
L5  10uH  WE-LQS-5040  [WE-LQS-5040]
LED7  BLUE  LED0603  [0603]
LED8  BLUE  LED0603  [0603]
LED9  BLUE  LED0603  [0603]
M10  NTS4173P  PCH_SOT323  [SOT323]
R72  10k  RR0603_BOX  [R0603_BOX]
R73  10k  RR0603_BOX  [R0603_BOX]
R74  10k  RR0603_BOX  [R0603_BOX]
R75  10k  RR0603_BOX  [R0603_BOX]
R76  10k  RR0603_BOX  [R0603_BOX]
R77  249  RR0603_BOX  [R0603_BOX]
R78  100k  RR0603_BOX  [R0603_BOX]
R79  100k  RR0603_BOX  [R0603_BOX]
R80  10k (x4)  R_ARRAY_4X_CRA06S  [R_VISHAY_CRA06S]
R81  10k  RR0603_BOX  [R0603_BOX]
R82  10k  RR0603_BOX  [R0603_BOX]
R83  30k  RR0603_BOX  [R0603_BOX]
R84  10m  SHUNT-LVK20  [LVK20]
R85  80.6k  RR0603_BOX  [R0603_BOX]
R86  16.5k  RR0603_BOX  [R0603_BOX]
R87  130k  RR0603_BOX  [R0603_BOX]
R88  182k  RR0603_BOX  [R0603_BOX]
R89  10k  RR0603_BOX  [R0603_BOX]
R90  10k  RR0603_BOX  [R0603_BOX]
R91  182k  RR0603_BOX  [R0603_BOX]
R92  30k  RR0603_BOX  [R0603_BOX]
R93  30k  RR0603_BOX  [R0603_BOX]
S1  JS202011CQN  SLIDE_SWITCH  [6-DPDT]
TP1  2501-2-00-80-00-00-07-0  TURRET_LARGE_2501  [TURRET_LARGE_2501]
TP2  2501-2-00-80-00-00-07-0  TURRET_LARGE_2501  [TURRET_LARGE_2501]
TP7  2501-2-00-80-00-00-07-0  TURRET_LARGE_2501  [TURRET_LARGE_2501]
TP8  2501-2-00-80-00-00-07-0  TURRET_LARGE_2501  [TURRET_LARGE_2501]
TP9  2501-2-00-80-00-00-07-0  TURRET_LARGE_2501  [TURRET_LARGE_2501]
TP10  2501-2-00-80-00-00-07-0  TURRET_LARGE_2501  [TURRET_LARGE_2501]
TP12  2501-2-00-80-00-00-07-0  TURRET_LARGE_2501  [TURRET_LARGE_2501]
TP13  2501-2-00-80-00-00-07-0  TURRET_LARGE_2501  [TURRET_LARGE_2501]
TP14  2308-2-00-80-00-00-07-0  TURRET_SMALL_2308  [TURRET_SMALL_2308]
U11  MCP23008-E/ML  [QFN20]
U12  LTC4313CMS8  [MSOP-8]
U13  24AA02T-I/OT  24AA64  [SOT-23-5]
U14  LT8471  [TSSOP20EXP]

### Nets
+3V3: C48.1 C50.1 M10.2(S) R72.1 R73.1 R74.1 R77.1 R80.R1_2 R80.R2_2 R80.R3_2 R80.R4_2 R81.1 U11.18 U12.8 ; also sheet 1,2,3
+12V: C54.1 C55.1 C58.2 L4.1 R84.I2 R85.2 R92.2 R93.2 TP14.TP1 U14.3(VIN1) U14.20(C2) ; also sheet 2
+12V_IN: C52.2 C53.+ J1.1 JP1.13 JP1.14 JP2.13 JP2.14 R78.1 R83.2 R84.I1 ; supply symbol labelled +12V ; also sheet 3
+15V: C55.2 C59.1 D3.C R88.2 U14.18(VIN2) ; also sheet 1
-15V: C60.2 D4.A R91.1 ; also sheet 1
A0_MUX: JP3.6 R80.R2_1 U11.3
A1_MUX: JP3.7 R80.R3_1 U11.2
A2_MUX: JP3.8 R80.R4_1 U11.1
ALERTB: JP1.3 JP2.3 TP10.TP ; also sheet 3
CTRL: C51.1 JP1.2 JP2.2 R82.2 S1.2(B:P) S1.5(A:P) ; also sheet 3
CTRL_P: R82.1 TP8.TP
EESCL: J2.11 R76.1 U13.1
EESDA: J2.12 R75.1 U13.3
FAULTB: JP1.1 JP2.1 TP9.TP ; also sheet 3
GND: C46.2 C47.2 C48.2 C49.2 C50.2 C51.2 C52.1 C53.- C54.2 C56.2 C57.2 C58.1 C59.2 C60.1 J1.2 J1.3 J2.3 J2.10 JP1.11 JP1.12 JP2.11 JP2.12 JP3.1 JP3.2 JP3.3 L5.1 LED7.C LED8.C LED9.C R79.2 R86.1 R87.1 R89.1 R90.2 S1.3(B:S) S1.6(A:S) TP1.TP TP2.TP U11.17 U11.PAD U12.4 U13.2 U13.5 U14.2(E1) U14.9(SYNC) U14.10(GND) U14.11(GND) U14.12(GND) U14.13(C3) U14.EXP(GND) ; also sheet 1,2,3
IIN_SNSM: R84.E2 ; also sheet 3
IIN_SNSP: R84.E1 ; also sheet 3
N$4: LED7.A R83.1
N$16: JP3.4 R81.2
N$42: D3.A L4.2 U14.1(C1)
N$44: R85.1 R86.2 U14.6(OV/UV)
N$46: C57.1 U14.15(SS2)
N$47: C56.1 U14.8(SS1)
N$48: R87.2 U14.7(RT)
N$50: D4.C L5.2 U14.19(E2)
N$51: M10.1(G) R78.2 R79.1
N$52: R90.1 R91.2 U14.16(FB2)
N$55: R88.1 R89.2 U14.5(FB1)
N$66: C49.1 R77.2 U11.4
N$74: R74.2 U11.9 U12.1
PG_+15V: LED8.A R92.1 U14.4(PG1)
PG_-15V: LED9.A R93.1 U14.17(PG2)
RESETB: JP1.7 JP2.7 ; also sheet 3
SCL: TP12.TP U12.2 ; also sheet 3
SCL_IN: J2.4 JP1.6 JP2.6 R73.2 U11.19 U12.3
SDA: TP13.TP U12.7 ; also sheet 3
SDA_IN: J2.2 JP1.4 JP2.4 R72.2 U11.20 U12.6
SHARE_CLK: JP1.5 JP2.5 JP3.5 TP7.TP ; also sheet 3
UNUSED1: JP1.9 JP2.9
UNUSED2: JP1.10 JP2.10
USB_3.3V: J2.5 M10.3(D)
USB_5V: C46.1 C47.1 J2.1 JP1.8 JP2.8 R75.2 R76.2 U13.4 ; supply symbol labelled +5V
Unconnected: J2.6 J2.7 J2.8 J2.9 R80.R1_1 S1.1(B:O) S1.4(A:O) U11.5 U11.6 U11.7 U11.8 U11.10 U11.11 U11.12 U11.13 U11.14 U11.15 U11.16 U12.5 U14.14(SHOUT)

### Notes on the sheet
- 1 | PRODUCTION | MIKE P. | 06-18-13
- POWER INPUT
- RUN | 9-14V
- (74404054068)
- OFF
- 1206
- 1206
- 1206
- 7343
- 1206
- (74404054100)
- PROVIDES Vin SUPPLIES FOR LDOs
- NOTE: UNLESS OTHERWISE SPECIFIED
  1. All resistors are 1% tolerance
- 1206
- MIKE P.
- MIKE P.
- HV & NEG VOLTAGE and CURRENT
- SENSING/SERVO'ING with LTC2975 PSM
- Identity EEPROM for LTpowerPlay | Powers LTC2975 from ribbon cable when Vin is off. | LTC2975
- DEMO CIRCUIT 2518A | 1

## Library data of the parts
C1-C52 C54-C62 = rcl:C: CAPACITOR, European symbol
C53 = rcl:CPOL-US: POLARIZED CAPACITOR, American symbol
D1-D4 = diode:SCHOTTKY-DIODE: Schottky Diode
D5 = diode:ZENER-DIODE: Z-Diode
D7 = diode:DIODE-: DIODE
J1 = power-jack:PJ-002A
J2 = kalin:CONN_DC1613: Connector for LT DC1613 USB Dongle
JP1 JP2 = pinhead_2mm:PINHD-2X07: PIN HEADER
JP3 = switch:TDA04H0SK1: Ultra-miniature Surface Mount Half-pitch DIP Switch
L1 = Wurth_Electronics_Midcom_Speedy_and_standard_magnetics:WE-MAPI: Package Style: WE-MAPI Shielded Power Inductor
L2-L5 = Wurth_Electronics_Midcom_Speedy_and_standard_magnetics:WE-LQS: Package Style: WE-LQS SMD Power Inductor
LED1-LED10 = led:LED: LED
M1 = transistor-fet:NCH-PCH_
M2 M4-M9 = transistor-fet:NCH_
M3 M10 = transistor-fet:PCH_
Q1-Q5 = transistor-small-signal:PNP
R1-R9 R11-R61 R63-R79 R81-R83 R85-R98 = resistor:R: RESISTOR, American symbol
R10 = resistor:R_ARRAY_2X_DIVIDER: RESISTOR ARRAY used as a divider
R62 R80 = resistor:R_ARRAY_4X_CRA06S: Thick Film Resistor Array
R84 = resistor-shunt:SHUNT: Shunt with Force/Sense
S1 = switch:SLIDE_SWITCH: SLIDE SWITCH C&K COMPONENTS, DPDT THRU HOLE 0.3A
SW1 SW2 = switch:SWITCH_PTS635: PTS635SL25 Surface Mount Tactile Switch
TP1-TP13 = testpad:TURRET_LARGE_2501: Large Test Turret Mill Max 2501
TP14 = testpad:TURRET_SMALL_2308: Small Test Turret Mill-Max 2308
TP15-TP31 = testpad:TESTPOINT: Test Point
U1 = linear-technology:LT3081: Adjustable 1.5A Single Resistor LDO with Monitors
U2 U6 = linear-technology:LTC6101: HV High Side Current Sense Amplifier in ThinSOT
U3 = linear-technology:LT3090: -36V, 600mA Negative Linear Regulator with Programmable Current Limit
U4 = linear-technology:LT6105: Extended Input Range Current Sense Amplifier (DFN6, MSOP8)
U5 = linear-technology:LT8330: Boost/SEPIC/Inverting Converter with 1A, 60V Switch
U7 = linear-technology:LT8580
U8 = linear-technology:LTC2054
U9 = linear-technology:LTC2975: 4-Ch Power System Manager with EEPROM and Input and Output Current Measurement (QFN64)
U10 = kalin:SN74LVC2G34: Dual Buffer Gate
U11 = microchip:MCP23008: I2C 8-pin IO Expander
U12 = linear-technology:LTC4313: 2-Wire Bus Buffers with High Noise Margin
U13 = kalin:24AA64: 64Kbit I2C Serial EEPROM in SOT-23-5
U14 = linear-technology:LT8471: Dual Multi-Topology DC/DC Converters w/ 2A Switch
U15 = linear-technology:LT6015
U$39-U$41 = supply1:KELVIN-CONNECT

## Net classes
1 HV: clearance 0.254 mm to class 0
